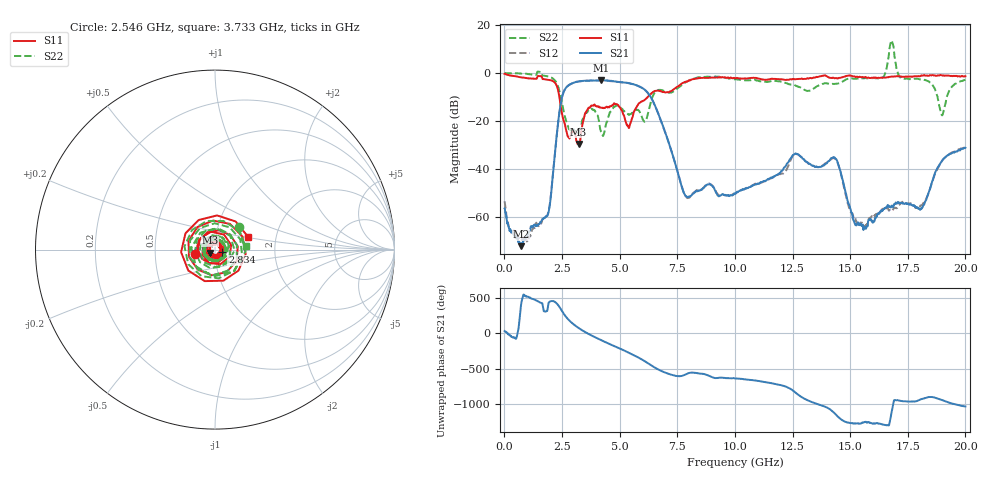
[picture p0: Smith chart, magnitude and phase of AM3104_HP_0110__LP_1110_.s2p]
!Created with skrf (http://scikit-rf.org).
# Hz S RI R 50.0
!freq ReS11 ImS11 ReS21 ImS21 ReS12 ImS12 ReS22 ImS22
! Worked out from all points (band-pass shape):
!   1601 points, 10 MHz to 20 GHz, reference 50 ohm
!   highest |S21| = -3.01 dB at 4.183 GHz (marker M1); lowest = -72.3 dB at 722.1 MHz (marker M2)
!   |S21| within 3 dB of the highest: 2.685 GHz to 5.939 GHz (3.253 GHz wide, 75.5 % of centre)
!   lowest |S11| = -29.6 dB at 3.221 GHz (marker M3), VSWR 1.07, Z = 47.2 - j1.58 ohm
!   |S11| at or under -10 dB: 2.384 GHz to 6.219 GHz (3.835 GHz wide, 89.1 % of centre)
!   |S22| runs from -26.3 to 13.6 dB; largest |S21 - S12| = 0.077
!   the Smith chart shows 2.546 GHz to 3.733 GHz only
!   S11 on the Smith chart (normalised r, x): 2.546 GHz: 0.80, -0.04; 2.834 GHz: 1.09, -0.03; 3.733 GHz: 1.44, +0.21
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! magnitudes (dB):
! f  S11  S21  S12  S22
! 10 MHz  -0.3  -56.6  -53.6  0.0
! 722.1 MHz  -1.8  -72.3  -69.9  -0.3
! 1.884 GHz  -2.8  -59.2  -58.8  -1.4
! 2.546 GHz  -19.1  -8.5  -8.6  -14.8
! 2.834 GHz  -27.2  -4.8  -4.8  -23.7
! 3.221 GHz  -29.6  -3.5  -3.6  -24.8
! 3.346 GHz  -24.0  -3.3  -3.4  -21.3
! 3.733 GHz  -14.1  -3.1  -3.2  -15.3
! 4.183 GHz  -14.5  -3.0  -3.0  -24.3
! 5.395 GHz  -23.0  -4.2  -4.2  -17.4
! 6.107 GHz  -11.0  -7.1  -7.2  -20.2
! 6.682 GHz  -7.3  -17.1  -17.1  -7.1
! 7.894 GHz  -3.7  -51.6  -51.9  -3.7
! 10.01 GHz  -2.2  -50.4  -50.4  -2.7
! 13.34 GHz  -2.2  -38.7  -38.6  -7.0
! 14.37 GHz  -2.1  -35.8  -36.0  -4.5
! 15.28 GHz  -1.5  -63.6  -62.2  -2.3
! 16.39 GHz  -1.9  -57.3  -56.9  -2.0
! 16.68 GHz  -1.6  -55.8  -57.5  7.3
! 18.11 GHz  -1.0  -56.6  -55.2  -2.7
! 18.98 GHz  -1.0  -36.8  -36.9  -17.6
! 20 GHz  -1.3  -31.3  -30.9  -2.9
